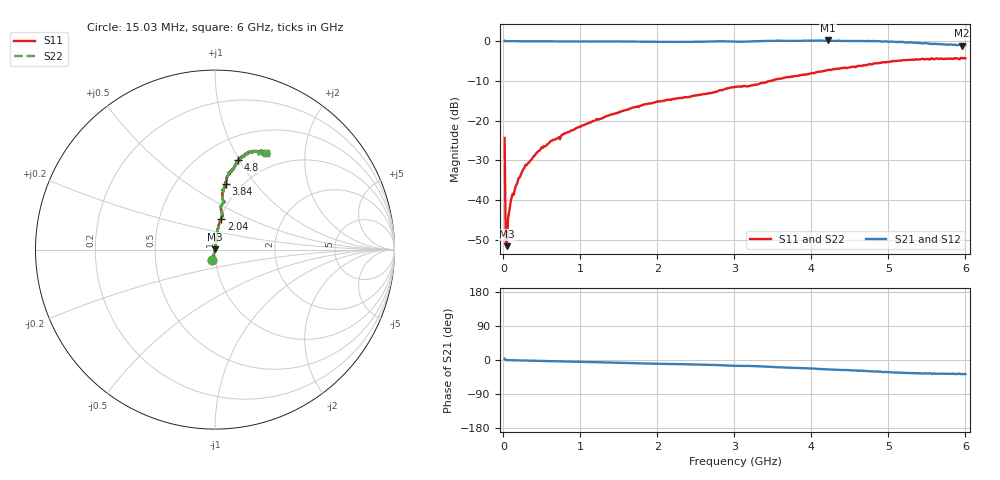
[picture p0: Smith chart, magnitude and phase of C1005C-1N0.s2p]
!	Network	Analyzer	HP8753E.07.74:	Oct	30	2002	Serial	No.	JP38451487
!	Hewlett-Packard
!	7	Sep	2009	8:16:31
!	Frequency	S11	S21	S12	S22
#	HZ	S	RI	R	50
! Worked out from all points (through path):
!   400 points, 15.03 MHz to 6 GHz, reference 50 ohm
!   highest |S21| = 0.17 dB at 4.215 GHz (marker M1); lowest = -1.1 dB at 5.955 GHz (marker M2)
!   group delay of S21, straight-line fit = 18.2 ps
!   lowest |S11| = -51.6 dB at 45.03 MHz (marker M3), VSWR 1.01, Z = 50.1 + j0.255 ohm
!   |S11| at or under -10 dB: start of sweep to 3.463 GHz
!   |S22| runs from -51.6 to -4.2 dB; largest |S21 - S12| = 0
!   S11 on the Smith chart (normalised r, x): 15.03 MHz: 0.96, -0.11; 2.04 GHz: 1.01, +0.36; 3.84 GHz: 0.85, +0.72; 4.8 GHz: 0.73, +0.99; 6 GHz: 0.78, +1.34
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1.502992e7  -0.0145 -0.0589  1.01 0.0589  1.01 0.0589  -0.0145 -0.0589
3.002985e7  0.00114 0.00279  0.999 -0.00279  0.999 -0.00279  0.00114 0.00279
4.502978e7  0.000674 0.00255  0.999 -0.00255  0.999 -0.00255  0.000674 0.00255
6.00297e7  0.00161 0.00578  0.998 -0.00578  0.998 -0.00578  0.00161 0.00578
1.050295e8  0.00192 0.0105  0.998 -0.0105  0.998 -0.0105  0.00192 0.0105
1.350293e8  0.00261 0.0114  0.997 -0.0114  0.997 -0.0114  0.00261 0.0114
1.95029e8  0.00214 0.0188  0.998 -0.0188  0.998 -0.0188  0.00214 0.0188
2.850286e8  0.0033 0.0275  0.997 -0.0275  0.997 -0.0275  0.0033 0.0275
4.950275e8  0.0041 0.0462  0.996 -0.0462  0.996 -0.0462  0.0041 0.0462
1.020025e9  0.0131 0.0852  0.987 -0.0852  0.987 -0.0852  0.0131 0.0852
2.01002e9  0.035 0.17  0.965 -0.17  0.965 -0.17  0.035 0.17
2.04002e9  0.0353 0.171  0.965 -0.171  0.965 -0.171  0.0353 0.171
3.015015e9  0.0474 0.263  0.953 -0.263  0.953 -0.263  0.0474 0.263
3.840011e9  0.0624 0.366  0.938 -0.366  0.938 -0.366  0.0624 0.366
4.00501e9  0.063 0.394  0.937 -0.394  0.937 -0.394  0.063 0.394
4.215009e9  0.0742 0.428  0.926 -0.428  0.926 -0.428  0.0742 0.428
4.800006e9  0.129 0.501  0.871 -0.501  0.871 -0.501  0.129 0.501
5.010005e9  0.164 0.523  0.836 -0.523  0.836 -0.523  0.164 0.523
5.565002e9  0.259 0.554  0.741 -0.554  0.741 -0.554  0.259 0.554
5.925e9  0.262 0.53  0.738 -0.53  0.738 -0.53  0.262 0.53
5.955e9  0.304 0.534  0.696 -0.534  0.696 -0.534  0.304 0.534
6e9  0.285 0.539  0.715 -0.539  0.715 -0.539  0.285 0.539
